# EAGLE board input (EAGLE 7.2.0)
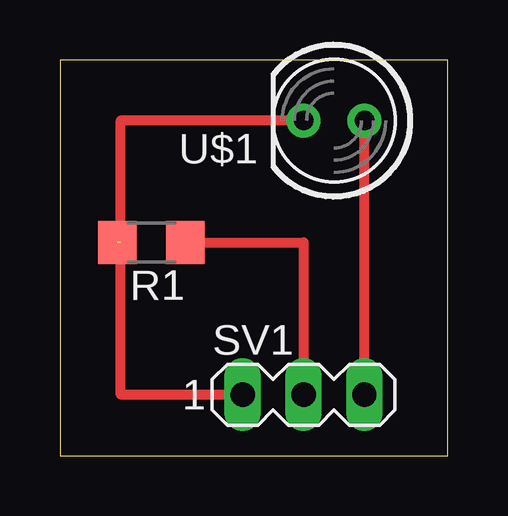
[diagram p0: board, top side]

Size 16.18 x 16.5 mm. Coordinates in mm from the lower left corner, seen from the top.
Outline: 0,0 16.18,0 16.18,16.5 0,16.5 0,0
Copper layers (1*16): Top 0.035mm / dielectric 1.5mm / Bottom 0.035mm
Design rules "default": minimum track width 10mil, minimum drill 24mil, track to track 8mil, track to pad 8mil, pad to pad 8mil, via to via 8mil, smd to smd 8mil, copper to edge 40mil, drill to drill 8mil, minimum pad ring 10mil, minimum via ring 8mil, stop-mask expansion 4mil, vias tented up to drill 0mil, thermal gap 10mil

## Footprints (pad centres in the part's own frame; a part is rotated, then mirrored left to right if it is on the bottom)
1206 = smd 1.6 x 1.803: 1 -1.422,0; 2 1.422,0
MA03-1 = drill 1.016 long: 1 -2.54,0; 2 0,0; 3 2.54,0
5MM = drill 0.813 pad 1.422: IN -1.27,0; OUT 1.27,0

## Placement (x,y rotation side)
R1  [1206]  3.81,8.89 180 top
SV1  [MA03-1]  10.16,2.54 0 top
U$1  [5MM]  11.43,13.97 180 top

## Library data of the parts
R1 U$1 = 01_FAB_Hello
SV1 = con-lstb; OC_FARNELL: unknown; OC_NEWARK: unknown

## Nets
GND: R1.1 SV1.2
PIN: R1.2 SV1.1 U$1.OUT
VCC: SV1.3 U$1.IN

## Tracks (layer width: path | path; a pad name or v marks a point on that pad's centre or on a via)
GND
  Top 0.406: R1.1 10.16,8.89 SV1.2
PIN  (1 unrouted)
  Top 0.406: R1.2 2.54,8.89 | 2.54,8.89 2.54,13.97 U$1.OUT | SV1.1 2.54,2.54 2.54,8.89
VCC
  Top 0.406: SV1.3 U$1.IN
